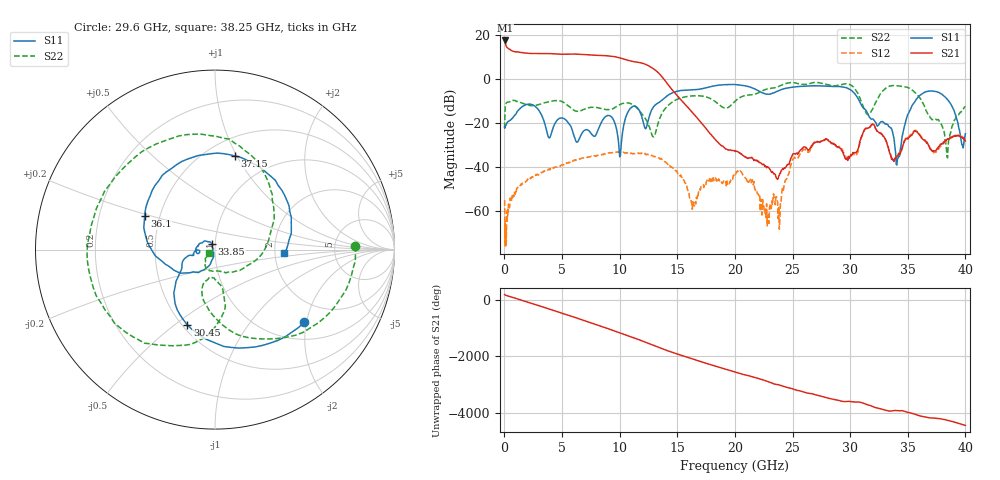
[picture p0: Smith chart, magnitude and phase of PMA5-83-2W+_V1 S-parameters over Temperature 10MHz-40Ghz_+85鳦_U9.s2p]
!Mini-Circuits Laboratory
!S-Parameters
!Model: US-AMP-1
!Run / Lot / Date Code: N/A / N/A / N/A
!Fixture: N/A, Pressing Arm: N/A
!Network Analyzer: NFA N8975A;  Serial number: 74408
!Date: 11/29/2023 at 10:19:53 AM
!No.: Unit# 2 (U9)
!Tested with: +85°C
! 2 port cal with Bias Tee PE1622 in line. No normalization applied. Bias cond 2: Vdd= 12V, Idd= 400mA, Vg2= 5V, starting point for Vg1= -2V
# Hz  S  dB  R  50
!Frequency  S11 dB  S11 Deg  S21 dB  S21 Deg  S12 dB  S12 Deg  S22 dB  S22 Deg
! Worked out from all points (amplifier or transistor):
!   826 points, 10 MHz to 40 GHz, reference 50 ohm
!   highest |S21| = 17.6 dB at 20 MHz (marker M1)
!   |S21| within 3 dB of that: start of sweep to 197.4 MHz
!   unconditionally stable (mu >= 1): start of sweep to end of sweep
!   at 5.6 GHz: K = 10.16, MAG = 11.7 dB, |S12| = -38.1 dB
!   at 19.4 GHz: K = 2181.48, MAG = -28.5 dB, |S12| = -48.1 dB
!   at 40 GHz: K = 285.17, MAG = -28.0 dB, |S12| = -27.4 dB
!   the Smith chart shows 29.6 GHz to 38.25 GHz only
!   S11 on the Smith chart (normalised r, x): 29.6 GHz: 1.42, -1.95; 30.45 GHz: 0.53, -0.56; 33.85 GHz: 0.96, +0.06; 36.1 GHz: 0.41, +0.19; 37.15 GHz: 0.68, +0.98; 38.25 GHz: 2.26, -0.11
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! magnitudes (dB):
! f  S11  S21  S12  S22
! 10 MHz  -22.0  17.3  -55.1  -22.4
! 20 MHz  -22.3  17.6  -59.2  -18.9
! 2.2 GHz  -11.4  11.7  -45.2  -12.0
! 6.7 GHz  -24.9  11.3  -36.1  -14.2
! 9.1 GHz  -16.6  10.5  -33.7  -13.9
! 10.05 GHz  -35.1  9.6  -33.4  -11.5
! 10.95 GHz  -13.2  8.2  -33.8  -11.2
! 12.25 GHz  -22.7  6.7  -34.1  -18.2
! 13.35 GHz  -10.8  2.9  -35.9  -19.8
! 16.4 GHz  -4.9  -15.8  -56.8  -7.7
! 20.05 GHz  -2.6  -33.0  -43.4  -9.9
! 22.75 GHz  -6.9  -40.4  -56.8  -4.6
! 26.7 GHz  -3.1  -30.2  -30.5  -1.7
! 29.6 GHz  -3.9  -36.2  -35.2  -2.1
! 30.45 GHz  -7.0  -33.6  -34.0  -4.7
! 31.9 GHz  -18.2  -20.6  -20.8  -14.1
! 33.35 GHz  -21.6  -32.0  -32.1  -3.4
! 33.85 GHz  -29.2  -36.4  -36.7  -2.9
! 36.1 GHz  -7.3  -26.1  -25.6  -9.0
! 37.15 GHz  -5.5  -32.8  -33.1  -18.5
! 38.25 GHz  -8.3  -27.7  -28.7  -27.6
! 40 GHz  -24.9  -28.2  -27.4  -12.4
